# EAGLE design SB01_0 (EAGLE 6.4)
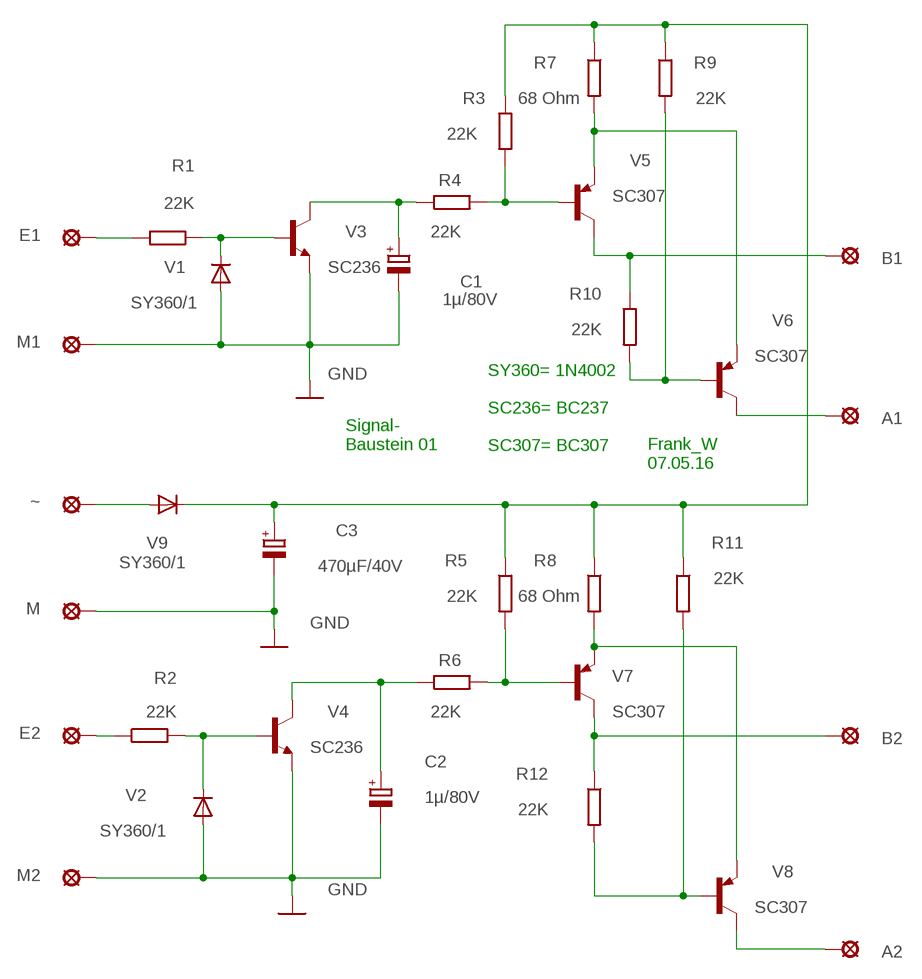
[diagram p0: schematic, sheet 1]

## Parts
A1  LSP10  [LSP10]
A2  LSP10  [LSP10]
B1  LSP10  [LSP10]
B2  LSP10  [LSP10]
C1  1µ/80V  CPOL-EUE5-5  [E5-5]
C2  1µ/80V  CPOL-EUE5-5  [E5-5]
C3  470µF/40V  CPOL-EUE22-9AXIAL  [E22-9]
E1  LSP10  [LSP10]
E2  LSP10  [LSP10]
M  LSP10  [LSP10]
M1  LSP10  [LSP10]
M2  LSP10  [LSP10]
R1  22K  R-EU_0207/12  [0207/12]
R2  22K  R-EU_0207/12  [0207/12]
R3  22K  R-EU_0207/12  [0207/12]
R4  22K  R-EU_0207/12  [0207/12]
R5  22K  R-EU_0207/12  [0207/12]
R6  22K  R-EU_0207/12  [0207/12]
R7  68 Ohm  R-EU_0207/12  [0207/12]
R8  68 Ohm  R-EU_0207/12  [0207/12]
R9  22K  R-EU_0207/12  [0207/12]
R10  22K  R-EU_0207/12  [0207/12]
R11  22K  R-EU_0207/12  [0207/12]
R12  22K  R-EU_0207/12  [0207/12]
V1  SY360/1  1N4004  [DO41-10]
V2  SY360/1  1N4004  [DO41-10]
V3  SC236  BC237  [TO92]
V4  SC236  BC237  [TO92]
V5  SC307  BC327  [TO92]
V6  SC307  BC327  [TO92]
V7  SC307  BC327  [TO92]
V8  SC307  BC327  [TO92]
V9  SY360/1  1N4004  [DO41-10]
~  LSP10  [LSP10]

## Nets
GND: C1.- C2.- C3.- M1.MP M2.MP M.MP V1.A V2.A V3.1(E) V4.1(E)
N$1: R1.1 V1.C V3.2(B)
N$2: R3.2 R4.2 V5.2(B)
N$3: C1.+ R4.1 V3.3(C)
N$4: R7.2 V5.1(E) V6.1(E)
N$5: B1.MP R10.1 V5.3(C)
N$6: R9.2 R10.2 V6.2(B)
N$7: A1.MP V6.3(C)
N$9: E2.MP R2.1
N$10: E1.MP R1.2
N$11: C3.+ R3.1 R5.1 R7.1 R8.1 R9.1 R11.1 V9.C
N$12: R2.2 V2.C V4.2(B)
N$13: C2.+ R6.1 V4.3(C)
N$14: R5.2 R6.2 V7.2(B)
N$15: R8.2 V7.1(E) V8.1(E)
N$16: B2.MP R12.1 V7.3(C)
N$17: A2.MP V8.3(C)
N$19: V9.A ~.MP
N$20: R11.2 R12.2 V8.2(B)

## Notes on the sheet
- SY360= 1N4002
  
  SC236= BC237
  
  SC307= BC307
- Signal-
  Baustein 01
- Frank_W
  07.05.16

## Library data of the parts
A1 A2 B1 B2 E1 E2 M M1 M2 ~ = solpad:LSP10: SOLDER PAD
C1-C3 = rcl:CPOL-EU: POLARIZED CAPACITOR, European symbol
R1-R12 = rcl:R-EU_: RESISTOR, European symbol
V1 V2 V9 = diode:1N4004: DIODE
V3 V4 = transistor-neu-to92:BC237: NPN TRANSISTOR
V5-V8 = transistor-pnp:BC327: PNP Transistor

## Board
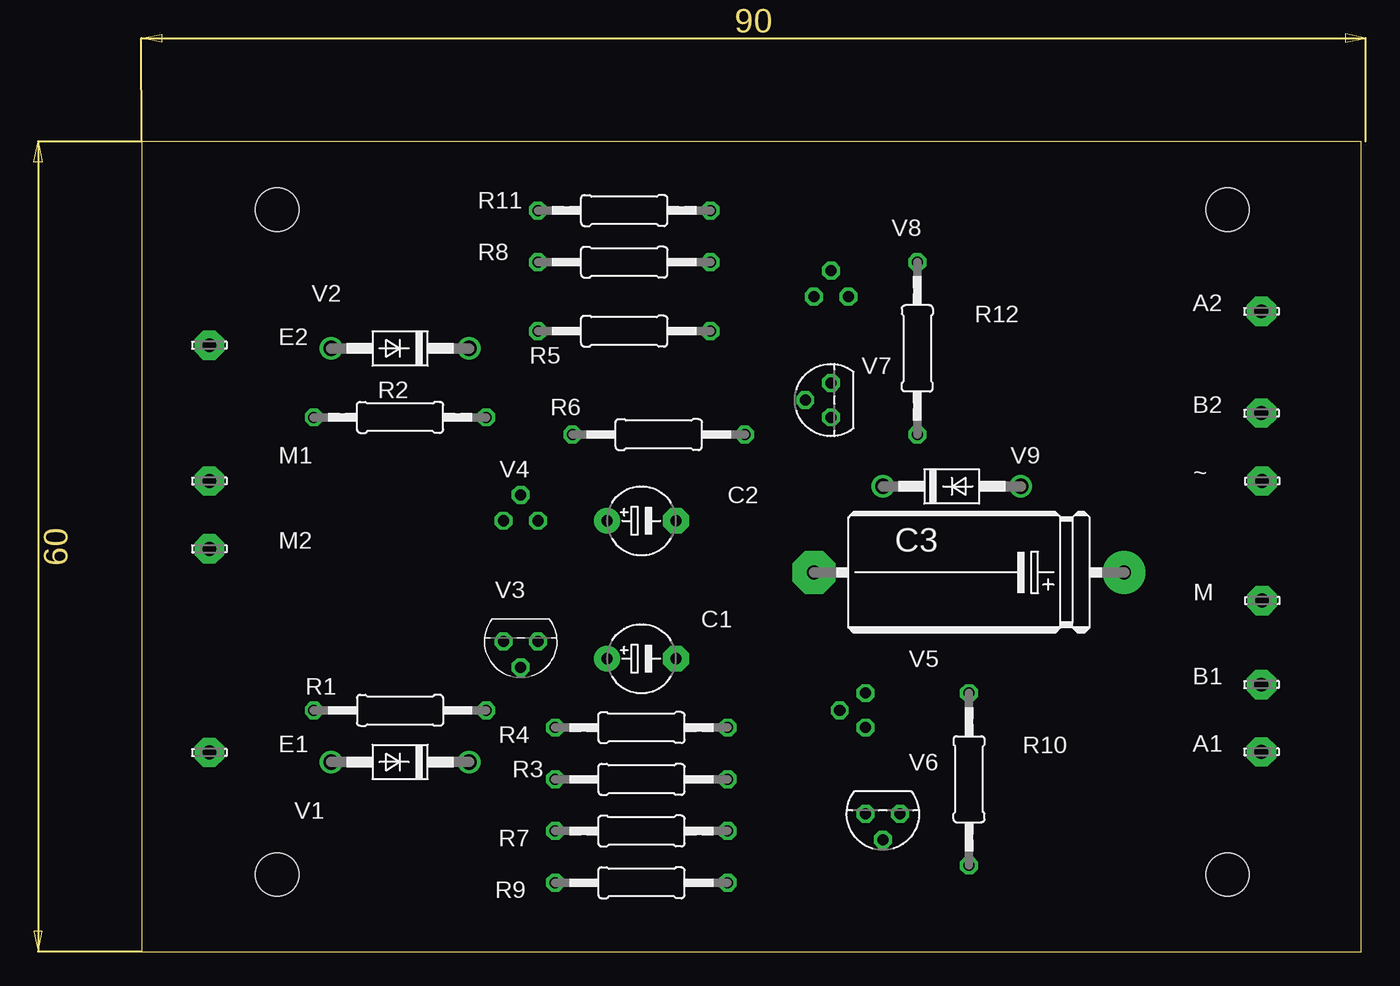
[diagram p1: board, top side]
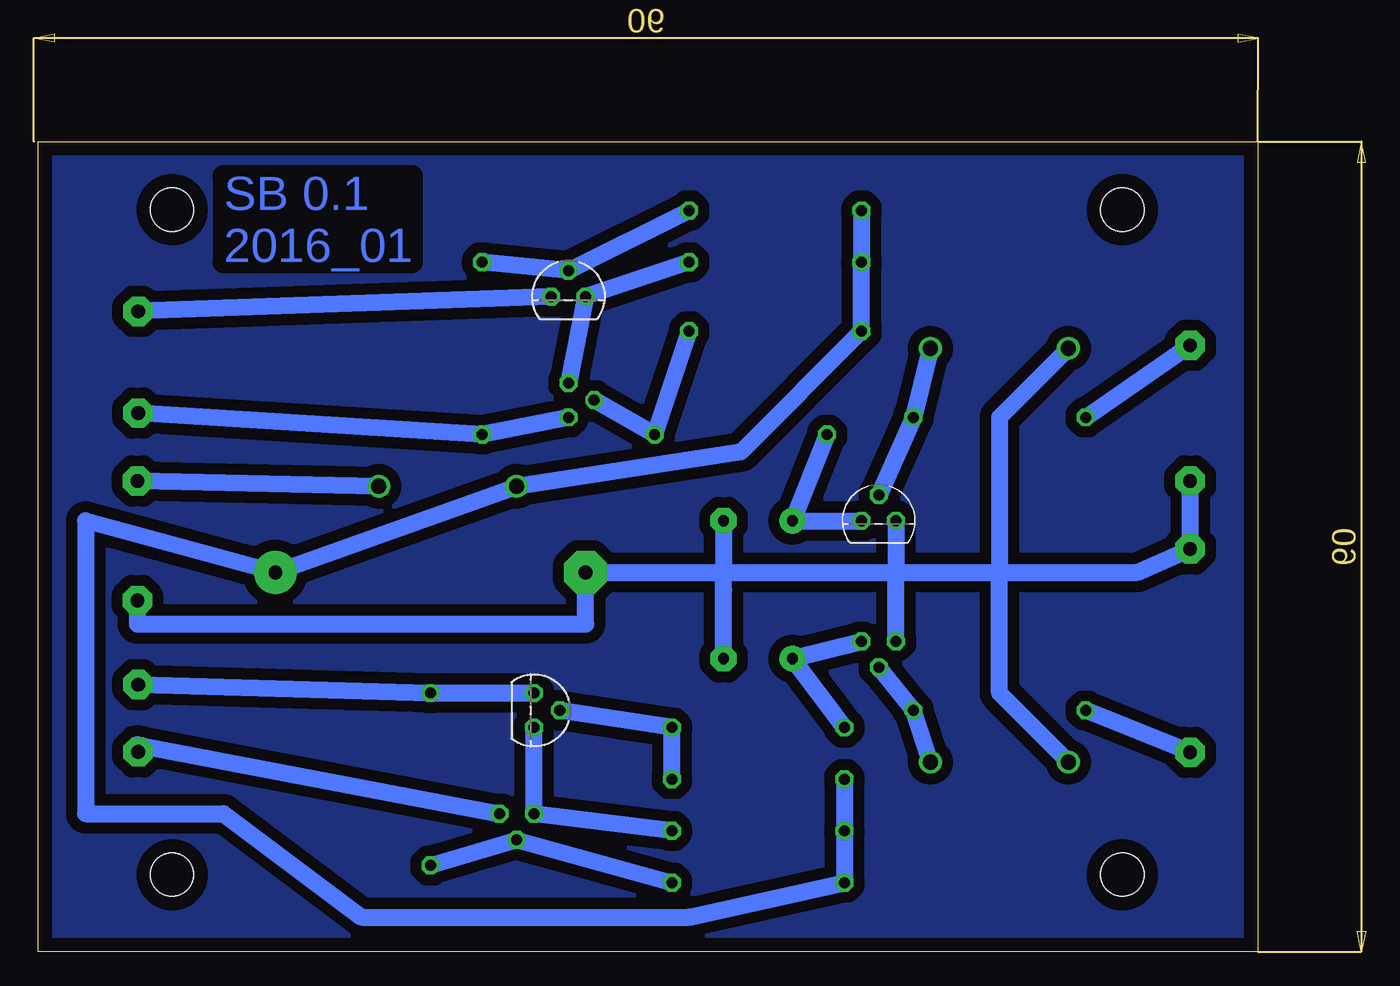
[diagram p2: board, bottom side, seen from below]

Size 98.09 x 67.61 mm. Coordinates in mm from the lower left corner, seen from the top.
Outline: 7.92,0 97.76,0 97.76,59.68 7.92,59.68 7.92,0
Copper layers (1*16): Top 0.035mm / dielectric 1.5mm / Bottom 0.035mm
Design rules "default *": minimum track width 20mil, minimum drill 24mil, track to track 8mil, track to pad 8mil, pad to pad 8mil, via to via 8mil, smd to smd 8mil, copper to edge 40mil, drill to drill 8mil, minimum pad ring 10mil, minimum via ring 8mil, stop-mask expansion 4mil, vias tented up to drill 0mil, thermal gap 20mil
Holes 3.2 mm at 87.92,54.68 87.92,5.68 17.92,5.68 17.92,54.68

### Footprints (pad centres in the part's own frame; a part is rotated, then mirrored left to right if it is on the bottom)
LSP10 = drill 1.016 pad 2.159 octagon: MP 0,0
E5-5 = drill 0.813 pad 1.905: + -2.54,0 | drill 0.813 pad 1.905 octagon: - 2.54,0
E22-9 = drill 1.016 pad 3.15: + -11.43,0 | drill 1.016 pad 3.15 octagon: - 11.43,0
0207/12 = drill 0.813 octagon: 1 -6.35,0; 2 6.35,0
DO41-10 = drill 1.118: A 5.08,0; C -5.08,0
TO92 = drill 0.813 octagon: 1 1.27,0; 2 0,1.905; 3 -1.27,0

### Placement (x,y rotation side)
A1  90.42,14.72 0 top
A2  90.42,47.18 0 top
B1  90.42,19.68 0 top
B2  90.42,39.68 0 top
C1  44.75,21.59 0 top
C2  44.75,31.75 0 top
C3  68.88,27.94 180 top
E1  12.92,14.68 0 top
E2  12.92,44.68 0 top
M  90.47,25.87 0 top
M1  12.92,34.68 0 top
M2  12.92,29.68 0 top
R1  26.97,17.78 180 top
R2  26.97,39.37 0 top
R3  44.75,12.7 0 top
R4  44.75,16.51 0 top
R5  43.48,45.72 0 top
R6  46.02,38.1 0 top
R7  44.75,8.89 0 top
R8  43.48,50.8 0 top
R9  44.75,5.08 0 top
R10  68.88,12.7 270 top
R11  43.48,54.61 0 top
R12  65.07,44.45 90 top
V1  26.97,13.97 180 top
V2  26.97,44.45 180 top
V3  35.86,22.86 180 top
V4  35.86,31.75 0 bottom
V5  61.26,17.78 270 bottom
V6  62.53,10.16 180 top
V7  58.72,40.64 90 top
V8  58.72,48.26 0 bottom
V9  67.61,34.29 0 top
~  90.47,34.68 0 top

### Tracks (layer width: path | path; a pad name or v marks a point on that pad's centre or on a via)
GND
  Bottom 1.27: M.MP 90.47,24.13 57.45,24.13 C3.- 47.29,27.94 | 47.29,27.94 34.59,27.94 | 34.59,27.94 26.97,27.94 | 26.97,27.94 16.81,27.94 M2.MP M1.MP | V1.A 26.97,19.05 26.97,27.94 | V4.1 34.59,27.94 | V3.1 34.59,27.94 | V2.A 26.97,39.37 26.97,27.94 | C1.- 47.29,26.67 47.29,27.94 | C2.- 47.29,27.94
N$1
  Bottom 1.27: V1.C R1.1 V3.2
N$2
  Bottom 1.27: R3.2 R4.2 V5.2
N$3
  Bottom 1.27: V3.3 C1.+ R4.1
N$4
  Bottom 1.27: V5.1 V6.1 R7.2
N$5
  Bottom 1.27: B1.MP R10.1 V5.3
N$6
  Bottom 1.27: R9.2 V6.2 R10.2
N$7
  Bottom 1.27: A1.MP 90.47,15.24 V6.3
N$8
  pour Bottom (isolate 0.813): 7.92,59.69 98.09,59.69 98.09,0 7.92,0
N$9
  Bottom 1.27: R2.1 E2.MP
N$10
  Bottom 1.27: E1.MP R1.2
N$11
  Bottom 1.27: R3.1 R7.1 R9.1 49.83,2.54 73.96,2.54 84.12,10.16 94.28,10.16 94.28,31.75 C3.+ V9.C 46.02,36.83 R5.1 R8.1 R11.1
N$12
  Bottom 1.27: V2.C R2.2 V4.2
N$13
  Bottom 1.27: V4.3 C2.+ R6.1
N$14
  Bottom 1.27: R5.2 R6.2 V7.2
N$15
  Bottom 1.27: R8.2 V8.1 V7.1
N$16
  Bottom 1.27: V7.3 R12.1 B2.MP
N$17
  Bottom 1.27: V8.3 A2.MP
N$19
  Bottom 1.27: V9.A ~.MP
N$20
  Bottom 1.27: R11.2 V8.2 R12.2

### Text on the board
Bottom: SB 0.1 / 2016_01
